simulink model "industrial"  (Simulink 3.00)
settings: Solver=ode45  StartTime=0.0  StopTime=3  RelTol=1e-8  AbsTol=1e-8

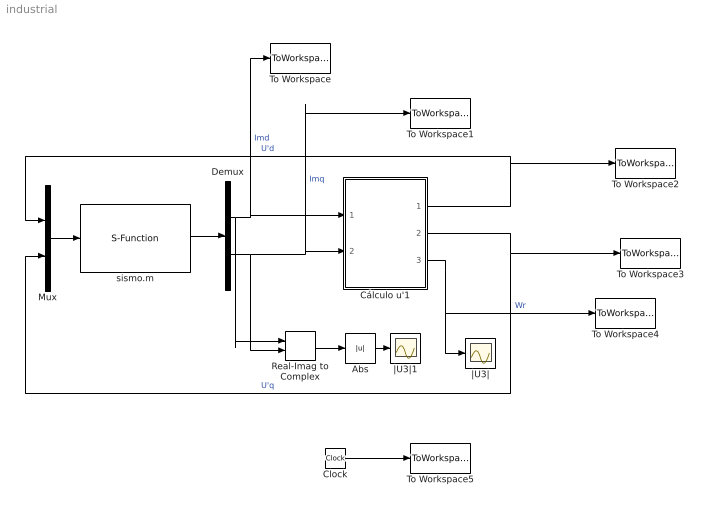
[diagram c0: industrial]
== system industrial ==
  Abs : Abs
  Clock : Clock
  Cálculo u'1 : Subsystem  mask(Modelo del rotor  del motor){Um=1, Pm=3, Am=1, Bm=0, Cm=0, Dm=0, Hm=5.8125, Xm=0.9806, Xr=0.043871, Rr=0.0023225, Xs=0.01729, Rs=0.0033548}
      mask prompts: Um "Tensión de alimentación (p.u)"; Pm "Potencia en el eje (p.u.)"; Am "Parámetro A modelo de Tcarga"; Bm "Parámetro B modelo de Tcarga"; Cm "Parámetro C modelo de Tcarga"; Dm "Parámetro D modelo de Tcarga"; Hm "Inercia,  H (s)"; Xm "Reactancia de Magnetización,  Xm (p.u.)"; Xr "Reactancia Rotor,  Xr  (p.u.)"; Rr "Resistencia del Rotor,  Rr  (p.u.)"; Xs "Reactancia del estator,  Xs  (p.u.)"; Rs "Resistencia del estator,  Rs  (p.u.)"
  Demux : Demux  Outputs=2
  Mux : Mux  Inputs=2
  Real-Imag to Complex : RealImagToComplex  Input=RealAndImag  ConstantPart=0
  To Workspace : ToWorkspace  VariableName=Id  SampleTime=-1  SaveFormat=Matrix
  To Workspace1 : ToWorkspace  VariableName=Iq  SampleTime=-1  SaveFormat=Matrix
  To Workspace2 : ToWorkspace  VariableName=Ud  SampleTime=-1  SaveFormat=Matrix
  To Workspace3 : ToWorkspace  VariableName=Uq  SampleTime=-1  SaveFormat=Matrix
  To Workspace4 : ToWorkspace  VariableName=Wr  SampleTime=-1  SaveFormat=Matrix
  To Workspace5 : ToWorkspace  VariableName=t  SampleTime=-1  SaveFormat=Matrix
  sismo.m : S-Function  FunctionName=sismo  Parameters=U1,gU1,Rsis,Xsis,Rs,Xs,Xm,Xr  PortCounts=[]  SFunctionModules=''  mask{U1=0.8, gU1=0, Rsis=0, Xsis=0.03118657106250, Rs=0.0033548, Xs=0.01729, Xm=0.9806, Xr=0.043871}
      mask prompts: U1 "Módulo de la tensión de alimentación [ pu. ]"; gU1 "Fase de la tensión de alimentación [ ° ]"; Rsis "Resistencia del Sistema Equivalente [ pu. ]"; Xsis "Reactancia del Sistema Equivalente [ pu. ]"; Rs "Resistencia del estator del motor [ pu. ]"; Xs "Reactancia del estator del motor [ pu. ]"; Xm "Reactancia de Magnetización del Motor [ pu. ]"; Xr "Reactancia del rotor del motor [ pu. ]"
  |U3| : Scope
  |U3|1 : Scope
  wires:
  Mux/1 -> sismo.m/1
  sismo.m/1 -> Demux/1
  Abs/1 -> |U3|1/1
  Real-Imag to Complex/1 -> Abs/1
  Demux/1 -> Real-Imag to Complex/1, Cálculo u'1/1(ids), To Workspace/1  "Imd"
  Demux/2 -> Real-Imag to Complex/2, Cálculo u'1/2(iqs), To Workspace1/1  "Imq"
  Cálculo u'1/1(u'd) -> Mux/1, To Workspace2/1  "U'd"
  Cálculo u'1/2(u'q) -> Mux/2, To Workspace3/1  "U'q"
  Cálculo u'1/3(wr) -> |U3|/1, To Workspace4/1  "Wr"
  Clock/1 -> To Workspace5/1

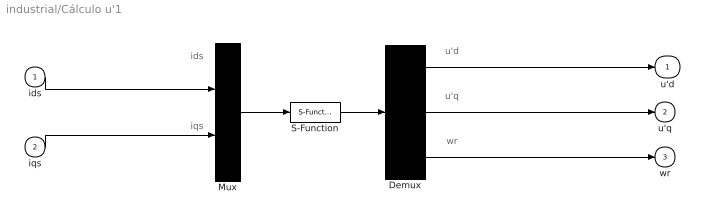
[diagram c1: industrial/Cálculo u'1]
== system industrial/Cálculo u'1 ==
  note: wr
  note: u'q
  note: u'd
  note: iqs
  note: ids
  ids : Inport  Port=1  PortWidth=-1  SampleTime=-1  DataType=auto
  iqs : Inport  Port=2  PortWidth=-1  SampleTime=-1  DataType=auto
  Demux : Demux  Outputs=3
  Mux : Mux  Inputs=2
  S-Function : S-Function  FunctionName=rotorind  Parameters=Rs, Xs, Rr, Xr, Xm, Hm, Am, Bm, Cm, Dm, Pm, Um  PortCounts=[]  SFunctionModules=''
  u'd : Outport  Port=1
  u'q : Outport  Port=2
  wr : Outport  Port=3
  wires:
  ids/1 -> Mux/1
  iqs/1 -> Mux/2
  S-Function/1 -> Demux/1
  Mux/1 -> S-Function/1
  Demux/1 -> u'd/1
  Demux/2 -> u'q/1
  Demux/3 -> wr/1
